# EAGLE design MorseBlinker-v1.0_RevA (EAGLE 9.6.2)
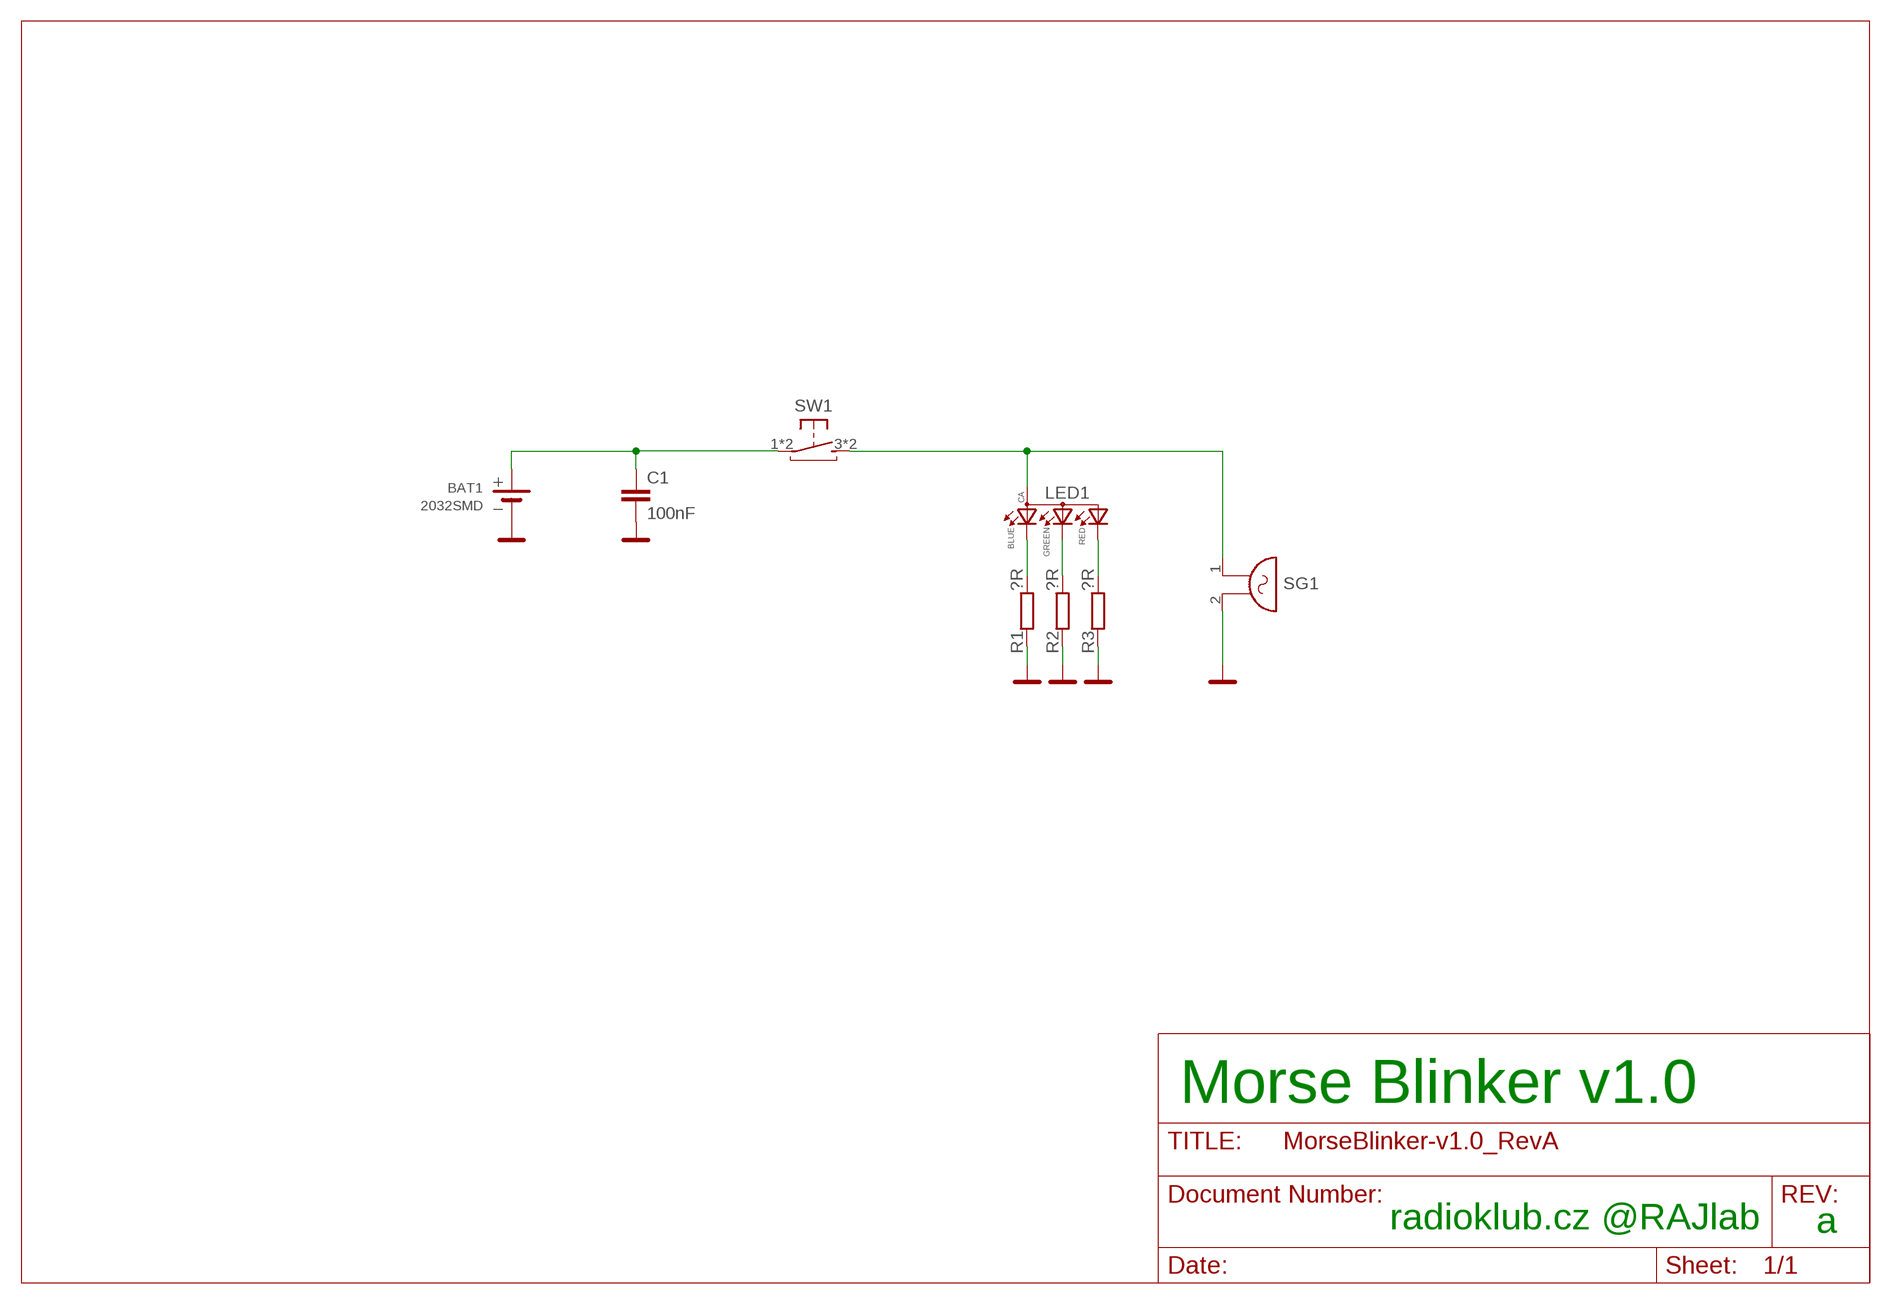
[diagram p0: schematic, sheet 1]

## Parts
BAT1  2032SMD  [DS1092-10-W6L_SMD]
C1  100nF  C-EUC0805  [C0805]
LED1  0.13_RGB_LEDPLCC  [P-LCC-4-3]
R1  ?R  R-EU_R0805  [R0805]
R2  ?R  R-EU_R0805  [R0805]
R3  ?R  R-EU_R0805  [R0805]
SG1  F/HGP  [F/HGP]
SW1  TACT-SW_BTNSMTJLC_6X6X4.5  [TACTSW_6X6X4.5_SMT]

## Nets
B: LED1.3(BLUE) R1.2
G: LED1.2(GREEN) R2.2
GND: BAT1.- C1.2 R1.1 R2.1 R3.1 SG1.2
N$2: LED1.4(ANODE) SG1.1 SW1.3(S) SW1.4(S)
N$5: BAT1.+ C1.1 SW1.1(P) SW1.2(P)
R: LED1.1(RED) R3.2

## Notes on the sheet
- Morse Blinker v1.0
- radioklub.cz @RAJlab | a

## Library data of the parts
BAT1 = #PaJa_31:2032: Battery 2032
C1 = rcl:C-EU: CAPACITOR, European symbol
LED1 = SparkFun-LED:0.13_RGB_LED: Everlight Red/Green/Blue LED 67-23/R6GHBHC-B01/2T || 67-23/R6GHBH-B01 Size 3.2*2.8*1.9mm Mounting Type SMD Full-Color LED PLCC4 Emitting Color Red/Green/Blue (620-625/530-535/470-475 nm) Chip Material AlGaInP/InGaN/InGaN Luminous Intensity 57-112/225-450/36-72 mcd Viewing Angle 120 deg Lens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; PROD_ID: DIO-12986
R1-R3 = rcl:R-EU_: RESISTOR, European symbol
SG1 = buzzer:F/HGP: BUZZER; OC_FARNELL: unknown; OC_NEWARK: unknown
SW1 = #Ondra2:TACT-SW_BTN; LCSC_PART: C127509

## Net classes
0 default: width 0.127 mm, drill 0.2 mm, clearance 0.127 mm

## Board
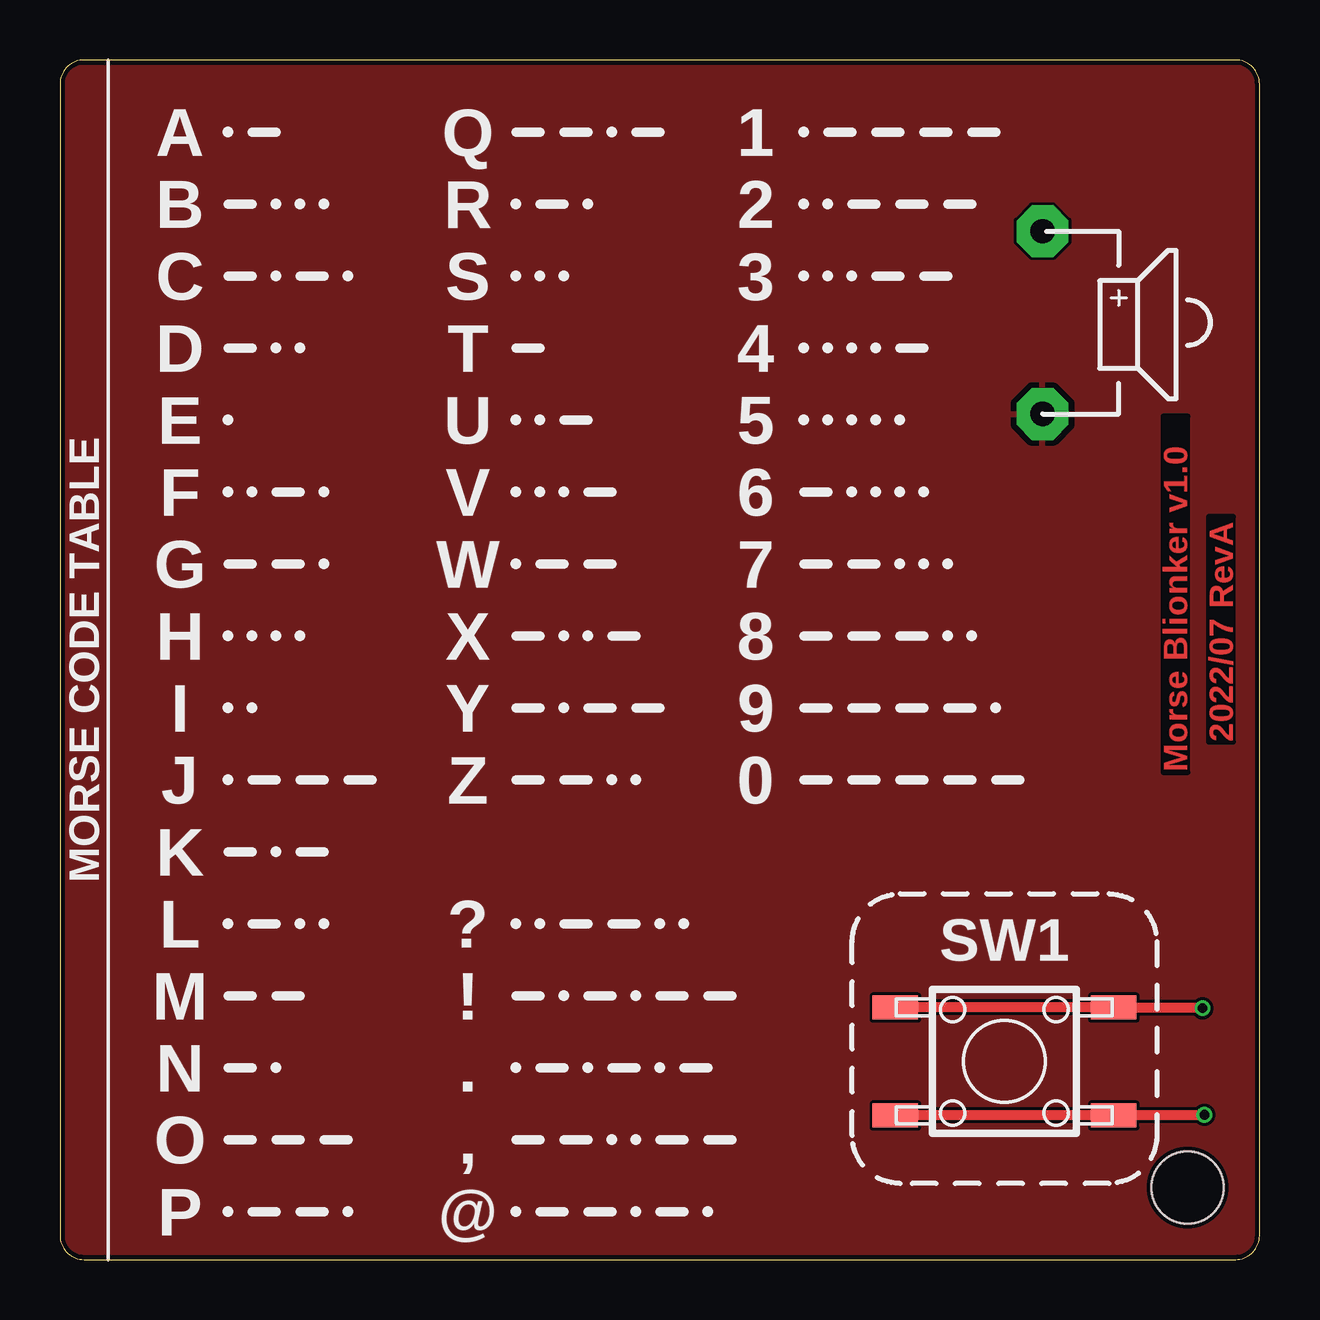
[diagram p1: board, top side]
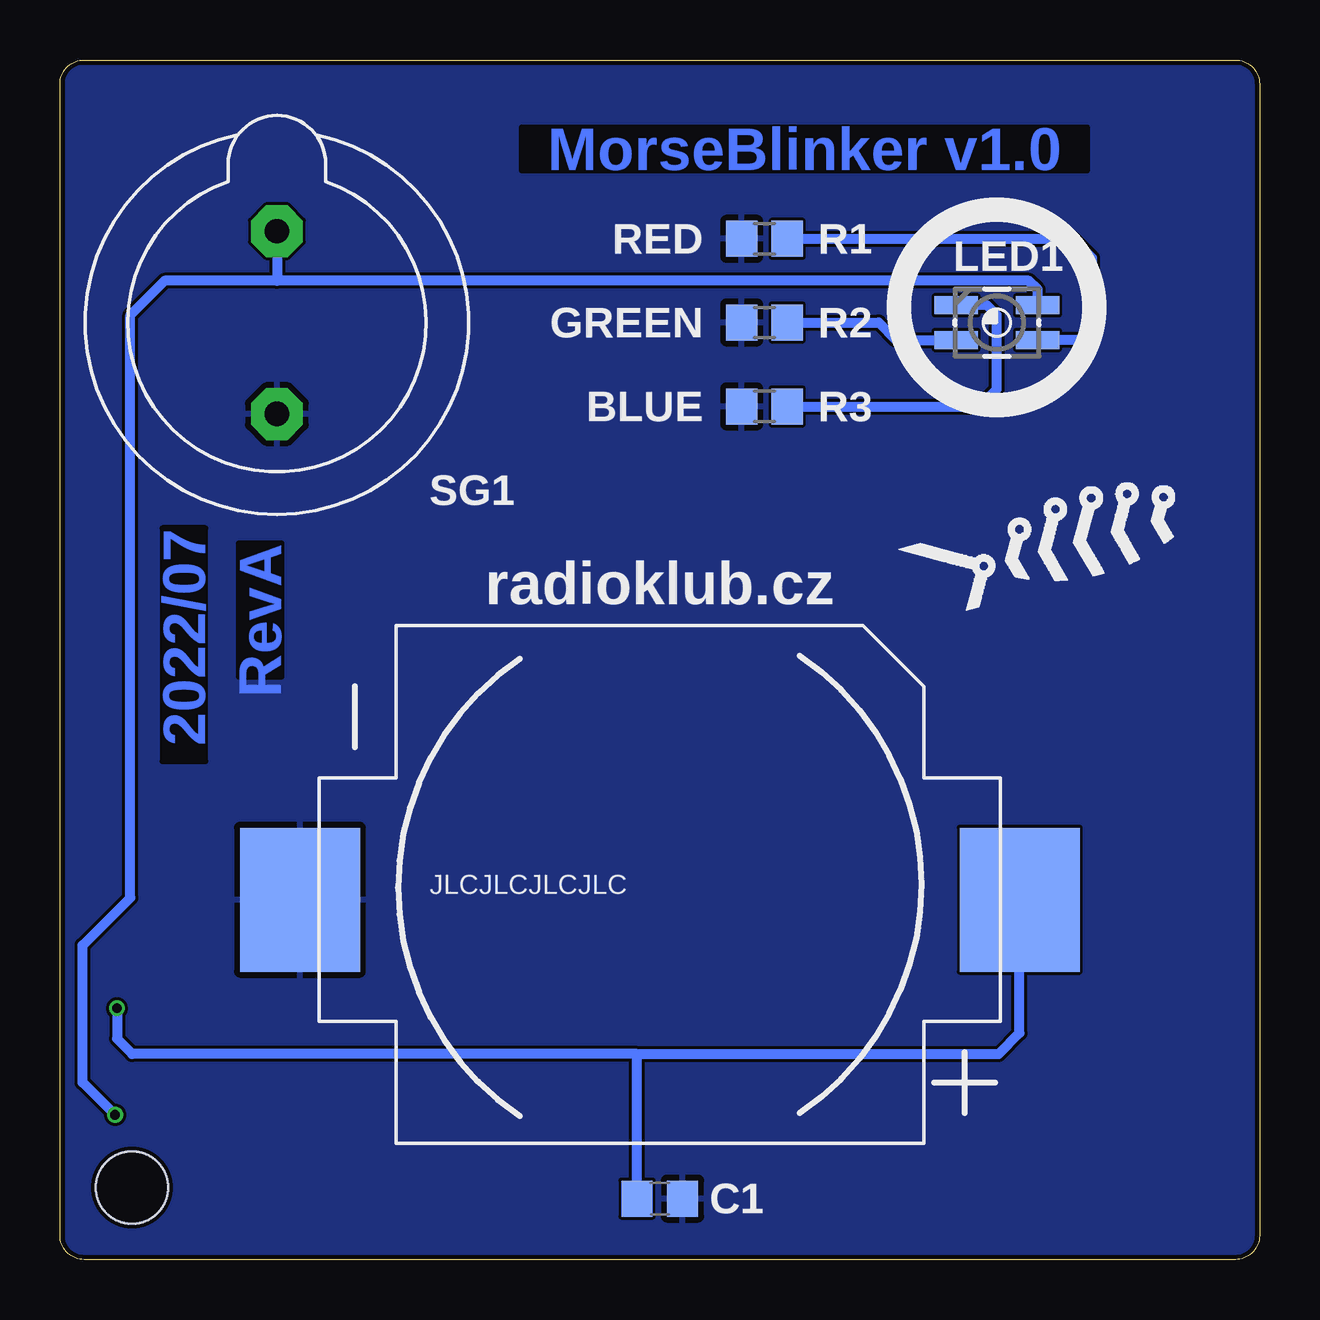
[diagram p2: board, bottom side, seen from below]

Size 50 x 50 mm. Coordinates in mm from the lower left corner, seen from the top.
Outline: 0,49 0,1 arc90 1,0 49,0 arc90 50,1 50,49 arc90 49,50 1,50 arc90 0,49
Copper layers (1*16): Top 0.035mm / dielectric 1.6mm / Bottom 0.035mm
Design rules "jlcpcb-2layers_od-Ondry3-assembly-tight": minimum track width 5mil, minimum drill 0.2mm, track to track 5mil, track to pad 5mil, pad to pad 5mil, via to via 5mil, smd to smd 5mil, copper to edge 0.2mm, drill to drill 6mil, minimum pad ring 0.13mm, minimum via ring 0.13mm, stop-mask expansion 4mil, vias tented up to drill 0.6mm, thermal gap 10mil
Holes 3 mm at 47,3

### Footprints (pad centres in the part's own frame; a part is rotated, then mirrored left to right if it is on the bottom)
DS1092-10-W6L_SMD = smd 5 x 6: + 15,0; - -15,0
C0805 = smd 1.3 x 1.5: 1 -0.95,0; 2 0.95,0
P-LCC-4-3 = smd 0.75 x 1.8: 1 0.725,1.7; 2 -0.725,1.7; 3 -0.725,-1.7; 4 0.725,-1.7
R0805 = smd 1.3 x 1.5: 1 -0.95,0; 2 0.95,0
F/HGP = drill 1.016 pad 2.159 octagon: 1 -3.81,0; 2 3.81,0
TACTSW_6X6X4.5_SMT = smd 1.9 x 1: 1 -4.55,2.25; 2 4.55,2.25; 3 -4.55,-2.25; 4 4.55,-2.25

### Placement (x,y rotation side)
BAT1  25,15 0 bottom
C1  25,2.54 0 bottom
LED1  10.95,39.05 90 bottom
R1  20.64,42.55 0 bottom
R2  20.64,39.05 0 bottom
R3  20.64,35.56 0 bottom
SG1  40.96,39.05 270 bottom
SW1  39.37,8.26 0 top
U$2  [RYBICKA_12MM]  7.62,29.84 0 bottom

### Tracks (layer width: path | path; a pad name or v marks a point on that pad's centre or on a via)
B
  Bottom 0.406: R1.2 7.78,42.55 6.99,41.75 6.99,38.73 7.39,38.33 LED1.3
G
  Bottom 0.406: R2.2 15.88,39.05 15.15,38.33 LED1.2
GND
  pour Bottom: 0,0 50.01,0 50.01,50.01 0,50.01
  pour Top: 0,0 0,50.01 50.01,50.01 50.01,0
N$2  (via drill 0.4)
  Top 0.406: v47.7,6.03 47.68,6 SW1.4 SW1.3
  Bottom 0.406: LED1.4 9.25,40.44 9.6,40.8 40.96,40.8 | 40.96,40.8 45.64,40.8 47.07,39.37 47.07,15.08 49.05,13.1 49.05,7.38 v47.7,6.03 | SG1.1 40.96,40.8
N$5  (via drill 0.4)
  Top 0.406: SW1.1 SW1.2 47.6,10.51 v47.62,10.48
  Bottom 0.406: v47.62,10.48 47.62,9.21 46.99,8.57 25.96,8.57 | BAT1.+ 10,15.64 10,9.45 10.87,8.57 25.96,8.57 | C1.1 25.95,8.57 25.96,8.57
R
  Bottom 0.406: R3.2 11.67,35.56 10.95,36.27 10.95,39.37 11.36,39.78 LED1.1

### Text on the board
Top: 2022/07 RevA | Morse Blionker v1.0
Bottom: MorseBlinker v1.0 | RevA | 2022/07
tPlace: A | Q | 1 | B | R | 2 | C | S | 3 | D | T | 4 | E | U | 5 | F | V | 6 | G | W | 7 | H | X | 8 | MORSE CODE TABLE | I | Y | 9 | J | Z | 0 | K | L | ? | M | ! | N | . | O | , | P | @
bPlace: JLCJLCJLCJLC
bNames: RED | GREEN | BLUE | radioklub.cz
bStop: MorseBlinker v1.0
